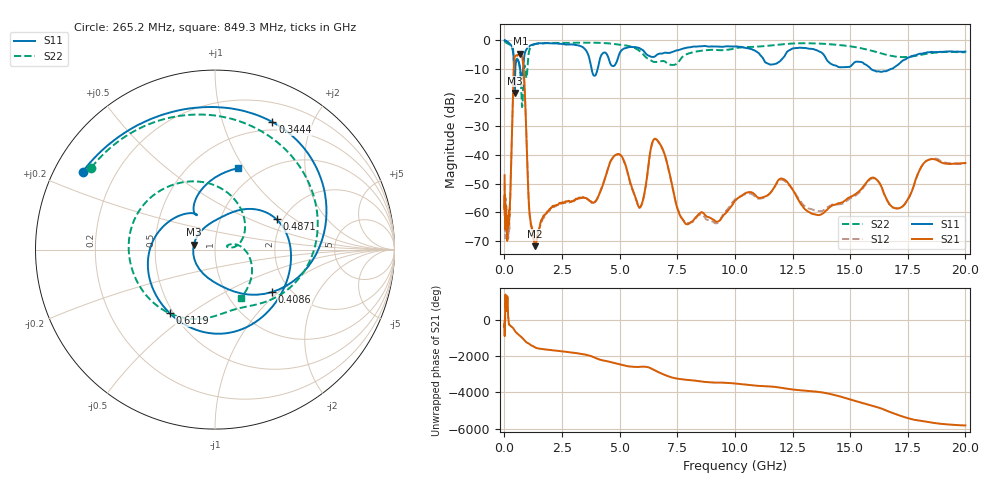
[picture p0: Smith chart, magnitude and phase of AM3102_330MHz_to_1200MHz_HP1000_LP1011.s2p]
! Date/Time: Tue, Sep 11, 2018 5:17 PM
! Network Analyzer: Agilent Technologies E8362B Rev: A.07.50.63
! Sweep from 0.010 to 20.000 GHz, 1601 Points, Sweep Type: LOG
! Power Supply: 4.949 V, 0.001 A
# Hz S DB R 50
!freq MagS11 AngS11 MagS21 AngS21 MagS12 AngS12 MagS22 AngS22
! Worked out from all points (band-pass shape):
!   1601 points, 10 MHz to 20 GHz, reference 50 ohm
!   highest |S21| = -4.66 dB at 692.3 MHz (marker M1); lowest = -71.8 dB at 1.327 GHz (marker M2)
!   |S21| within 3 dB of the highest: 422.2 MHz to 808.8 MHz (386.6 MHz wide, 62.8 % of centre)
!   lowest |S11| = -18.3 dB at 440.9 MHz (marker M3), VSWR 1.28, Z = 39.4 + j2.24 ohm
!   |S11| at or under -10 dB: 684.6 MHz to 812.4 MHz (127.8 MHz wide, 17.1 % of centre); 3.787 GHz to 4.044 GHz (256.9 MHz wide, 6.56 % of centre); 15.91 GHz to 16.77 GHz (854.9 MHz wide, 5.23 % of centre)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
!   |S22| runs from -23.2 to -0.2 dB; largest |S21 - S12| = 0.01
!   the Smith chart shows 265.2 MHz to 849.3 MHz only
!   S11 on the Smith chart (normalised r, x): 265.2 MHz: 0.08, +0.27; 344.4 MHz: 0.41, +1.47; 408.6 MHz: 1.61, -0.90; 487.1 MHz: 1.86, +0.73; 611.9 MHz: 0.48, -0.42; 849.3 MHz: 0.81, +0.94
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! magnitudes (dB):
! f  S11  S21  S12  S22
! 10 MHz  0.0  -47.1  -49.9  -0.2
! 35.55 MHz  0.0  -61.8  -63.3  -0.5
! 126.4 MHz  -0.4  -67.3  -65.5  -1.0
! 265.2 MHz  -1.4  -52.2  -51.4  -1.7
! 344.4 MHz  -2.2  -27.7  -27.8  -2.9
! 408.6 MHz  -8.1  -9.9  -9.9  -6.6
! 440.9 MHz  -18.3  -6.0  -6.1  -9.1
! 447.2 MHz  -17.8  -5.7  -5.8  -9.1
! 487.1 MHz  -8.4  -5.3  -5.4  -7.4
! 611.9 MHz  -7.2  -4.9  -5.0  -7.1
! 692.3 MHz  -10.5  -4.7  -4.7  -11.5
! 772.3 MHz  -13.0  -5.7  -5.7  -23.2
! 849.3 MHz  -6.5  -12.0  -12.1  -10.3
! 1.082 GHz  -2.0  -59.4  -60.1  -3.5
! 1.327 GHz  -1.2  -71.8  -71.1  -1.3
! 1.59 GHz  -1.0  -62.8  -63.6  -1.0
! 3.921 GHz  -12.3  -56.3  -56.4  -0.8
! 4.878 GHz  -7.3  -39.7  -39.8  -1.4
! 5.652 GHz  -2.3  -53.9  -54.3  -2.6
! 6.58 GHz  -5.2  -34.4  -34.5  -7.5
! 7.958 GHz  -2.5  -64.1  -63.7  -4.6
! 20 GHz  -3.9  -42.7  -43.3  -4.1
